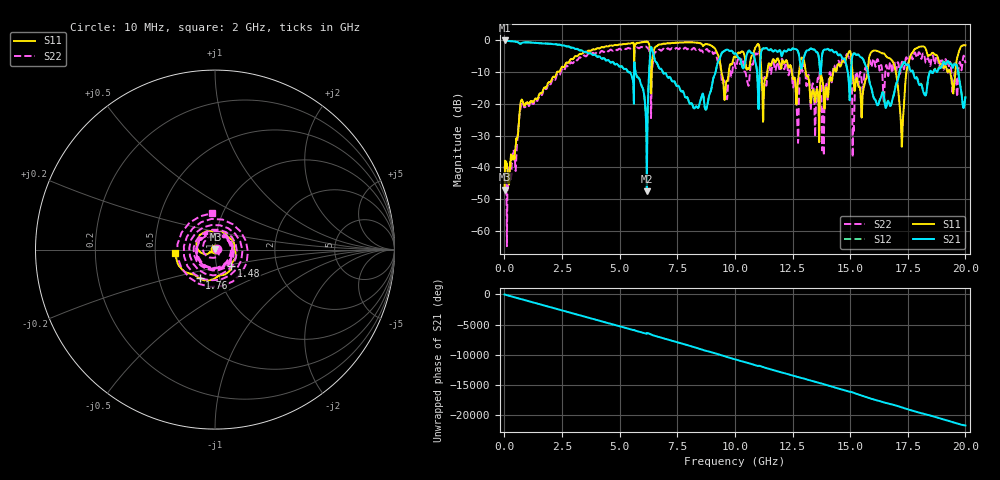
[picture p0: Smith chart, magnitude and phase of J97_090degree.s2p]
!Keysight Technologies,N5222A,MY51421036,A.10.65.16
!Date: Friday, March 31, 2023 14:31:22
!Correction: S11(Full 2 Port(1,2))
!S21(Full 2 Port(1,2))
!S12(Full 2 Port(1,2))
!S22(Full 2 Port(1,2))
!S2P File: Measurements: S11, S21, S12, S22:
# Hz S  dB  R 50
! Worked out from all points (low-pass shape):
!   2000 points, 10 MHz to 20 GHz, reference 50 ohm
!   highest |S21| = -0.01 dB at 10 MHz (marker M1); lowest = -47.5 dB at 6.18 GHz (marker M2)
!   |S21| within 3 dB of the highest: start of sweep to 3.231 GHz; 11.17 GHz to 11.45 GHz (286.7 MHz wide, 2.54 % of centre)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
!   lowest |S11| = -46.9 dB at 10 MHz (marker M3), VSWR 1.01, Z = 50.2 + j0.387 ohm
!   |S11| at or under -10 dB: start of sweep to 2.283 GHz; 13.07 GHz to 14.26 GHz (1.191 GHz wide, 8.71 % of centre); 15.1 GHz to 15.75 GHz (652.6 MHz wide, 4.23 % of centre)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
!   |S22| runs from -64.8 to -1.9 dB; largest |S21 - S12| = 0.021
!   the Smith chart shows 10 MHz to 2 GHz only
!   S11 on the Smith chart (normalised r, x): 10 MHz: 1.00, +0.01; 1.48 GHz: 1.18, -0.22; 1.76 GHz: 0.80, -0.27; 2 GHz: 0.64, -0.03
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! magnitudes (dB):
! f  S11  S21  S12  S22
! 10 MHz  -46.9  0.0  -0.1  -39.5
! 750 MHz  -18.6  -0.8  -0.8  -19.4
! 1.48 GHz  -17.7  -0.9  -0.8  -18.3
! 1.76 GHz  -14.8  -1.0  -1.0  -15.1
! 2 GHz  -13.1  -1.0  -1.0  -13.8
! 3.35 GHz  -4.2  -3.1  -3.1  -5.6
! 6.18 GHz  -0.4  -47.5  -47.4  -2.1
! 6.38 GHz  -13.1  -2.2  -2.1  -15.7
! 6.68 GHz  -1.4  -8.3  -8.2  -3.1
! 8.32 GHz  -0.7  -20.8  -20.7  -3.0
! 9.59 GHz  -15.3  -3.1  -3.1  -14.5
! 10.01 GHz  -5.1  -4.0  -4.1  -8.0
! 11.27 GHz  -14.7  -2.5  -2.5  -11.7
! 12.13 GHz  -7.0  -3.3  -3.3  -8.9
! 12.7 GHz  -16.6  -3.0  -2.9  -24.9
! 12.93 GHz  -5.5  -7.2  -7.2  -9.8
! 13.34 GHz  -17.1  -2.7  -2.7  -15.4
! 16.67 GHz  -5.5  -19.3  -19.2  -10.4
! 17.24 GHz  -33.5  -8.1  -8.0  -6.9
! 17.75 GHz  -3.3  -10.5  -10.4  -4.9
! 19.46 GHz  -16.3  -8.6  -8.3  -15.3
! 20 GHz  -1.6  -18.0  -17.6  -7.2
